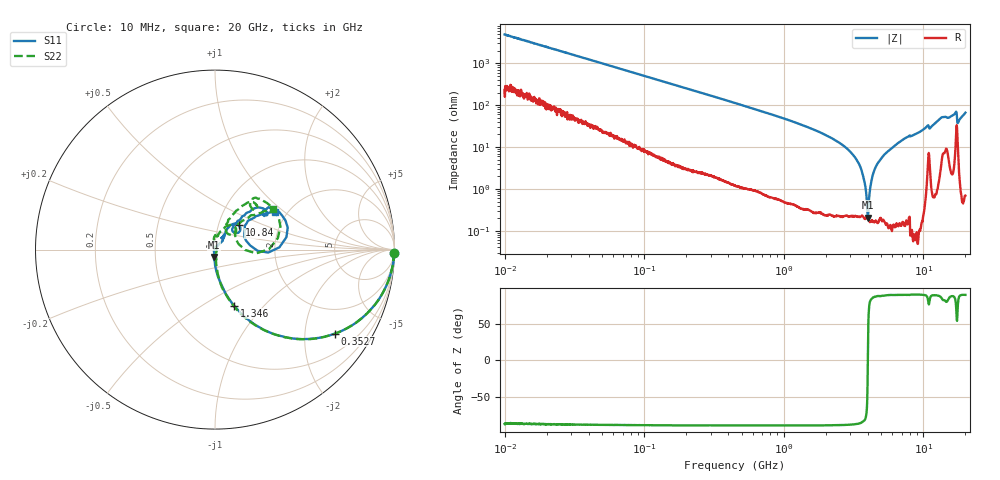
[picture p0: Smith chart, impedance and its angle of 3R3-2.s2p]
!Keysight Technologies,P5008B,MY61100088,A.16.20.02
!Date: Friday, August 30, 2024 11:26:35
!Correction: S11(C  2-Port  )
!S21(C  2-Port  )
!S12(C  2-Port  )
!S22(C  2-Port  )
!S2P File: Measurements: S11, S21, S12, S22:Log Frequency Sweep
# Hz S  dB  R 50
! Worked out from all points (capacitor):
!   1601 points, 10 MHz to 20 GHz, reference 50 ohm
!   read as one part in series: C = 3.26 pF near 10.39 MHz
!   lowest |Z| = 208 mohm at 3.996 GHz (marker M1)
!   series resonance near 4 GHz, so ESL is about 490 pH
!   S11 on the Smith chart (normalised r, x): 10 MHz: 3, -96; 352.7 MHz: 1.02, -2.85; 1.346 GHz: 0.99, -0.70; 10.84 GHz: 1.25, +0.35; 20 GHz: 1.73, +0.86
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1e7  -0.01 -1.2  -33.79 86.1  -33.79 86.1  -0.01 -1.2
3.555162e7  -0.04 -4.1  -22.94 84.2  -22.94 84.2  -0.04 -4.1
1.263918e8  -0.29 -14.1  -12.33 75.1  -12.34 75.1  -0.29 -14.1
3.526613e8  -1.76 -34.9  -4.92 54.4  -4.92 54.4  -1.76 -35.0
4.472136e8  -2.55 -41.6  -3.63 47.7  -3.63 47.7  -2.55 -41.7
1.34637e9  -9.65 -71.3  -0.53 18.0  -0.53 17.9  -9.65 -71.8
1.589917e9  -11.25 -74.9  -0.36 14.3  -0.37 14.3  -11.24 -75.3
2.865525e9  -18.62 -86.8  -0.08 3.4  -0.08 3.4  -18.53 -84.2
3.995989e9  -27.79 -96.4  -0.02 -2.3  -0.02 -2.4  -27.33 -81.8
4.786562e9  -39.22 -125.1  -0.01 -5.6  -0.01 -5.7  -37.35 -51.0
5.189161e9  -49.28 145.1  -0.00 -7.1  -0.01 -7.2  -40.82 7.9
5.652411e9  -39.39 71.6  -0.00 -8.8  -0.00 -8.8  -37.64 70.5
6.335038e9  -29.11 54.1  0.00 -11.1  0.00 -11.1  -28.97 92.6
7.066454e9  -24.13 48.7  -0.00 -13.5  -0.01 -13.6  -24.38 96.4
7.697294e9  -21.52 57.8  -0.02 -15.6  -0.02 -15.7  -21.74 85.6
8.750704e9  -21.94 60.4  -0.01 -18.9  -0.01 -19.0  -21.96 77.4
1.083639e10  -14.43 45.6  -0.56 -27.1  -0.56 -27.2  -15.65 44.4
1.147208e10  -15.60 51.9  -0.15 -27.0  -0.15 -27.1  -15.99 65.5
1.348308e10  -9.17 41.9  -0.81 -35.9  -0.82 -36.1  -9.41 51.2
1.661757e10  -8.07 35.4  -0.96 -44.4  -0.96 -44.6  -8.36 45.4
1.810106e10  -13.47 38.6  -0.33 -41.1  -0.34 -41.3  -13.95 47.1
2e10  -8.08 32.3  -0.75 -55.1  -0.75 -55.3  -8.11 35.3
